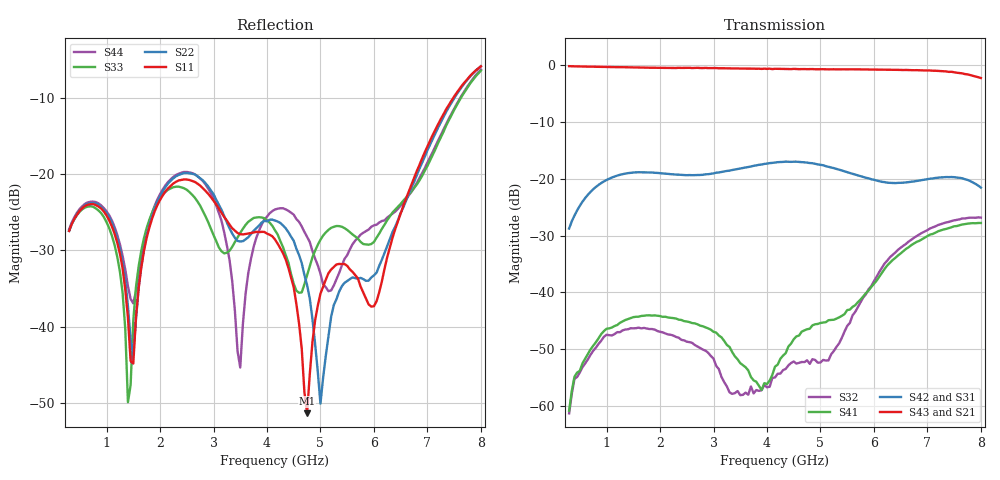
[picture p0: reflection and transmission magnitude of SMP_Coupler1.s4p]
! Created Sat Oct 21 10:14:57 2017
# hz S ma R 50
! 4 Port Network Data from SP1.SP block
! freq  magS11  angS11  magS12  angS12  magS13  angS13  magS14  angS14
!  magS21  angS21  magS22  angS22  magS23  angS23  magS24  angS24
!  magS31  angS31  magS32  angS32  magS33  angS33  magS34  angS34
!  magS41  angS41  magS42  angS42  magS43  angS43  magS44  angS44
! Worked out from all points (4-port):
!   155 points, 300 MHz to 8 GHz, reference 50 ohm
!   strongest paths, dB at 300 MHz, 2.2 GHz, 4.15 GHz, 6.1 GHz, 8 GHz:
!     S43: -0.1, -0.5, -0.6, -0.7, -2.2
!     S21: -0.1, -0.5, -0.6, -0.7, -2.4
!     S42: -28.8, -19.2, -17.1, -20.4, -21.6
!     S31: -28.8, -19.2, -17.1, -20.3, -21.0
!     S41: -60.9, -44.5, -53.1, -37.3, -27.8
!     S32: -61.4, -47.5, -55.0, -36.4, -26.8
!   lowest |S11| = -51.4 dB at 4.75 GHz (marker M1), VSWR 1.01, Z = 49.7 - j0.0107 ohm
!   |S11| at or under -10 dB: start of sweep to 7.481 GHz
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3e8  0.04244 27.7  0.9831 -40.6  0.03636 48.3  0.0009341 115.9
     0.9838 -40.4  0.04276 28.2  0.0008734 116.6  0.03641 48.6
     0.0363 48.6  0.0008558 114.7  0.0424 29.4  0.9844 -40.4
     0.0009028 116.1  0.03646 48.7  0.9841 -40.4  0.04352 27.7
1.3e9  0.02411 -120.5  0.9631 -173.1  0.11 -82.8  0.005552 -120.0
       0.9638 -173.1  0.02633 -125.2  0.004587 -121.2  0.1099 -83.3
       0.11 -82.8  0.004608 -121.1  0.01668 -111.2  0.9629 -172.7
       0.005533 -120.5  0.1099 -83.2  0.9637 -172.7  0.02914 -139.8
2.65e9  0.08906 -110.6  0.948 8.3  0.1076 99.9  0.005273 -23.3
        0.9498 8.4  0.09961 -116.2  0.003448 -7.6  0.1076 98.5
        0.1075 99.7  0.003423 -7.8  0.07016 -101.8  0.9478 9.2
        0.005314 -23.2  0.1077 98.7  0.9495 9.4  0.1001 -127.6
3.45e9  0.04116 -161.4  0.9392 -98.4  0.121 -6.7  0.002487 171.6
        0.9396 -98.3  0.03649 -164.6  0.001295 -108.4  0.1216 -9.2
        0.1208 -6.9  0.001345 -108.3  0.03842 -98.4  0.9367 -97.2
        0.002563 169.4  0.1219 -9.3  0.9399 -97.2  0.006884 69.4
4.75e9  0.002694 -177.7  0.9246 87.9  0.1384 -179.9  0.004856 165.2
        0.925 87.9  0.01875 106.9  0.002403 130.0  0.1385 177.6
        0.1382 -179.9  0.002511 127.8  0.02168 -114.7  0.9243 89.6
        0.004717 162.9  0.1388 177.7  0.9259 89.5  0.03883 104.9
6e9  0.0136 145.7  0.9199 -81.7  0.1005 12.0  0.01167 -1.8
     0.9215 -81.7  0.02167 161.0  0.01263 16.2  0.09824 6.6
     0.1001 11.9  0.01251 15.9  0.03591 -162.8  0.9203 -79.5
     0.01186 -1.9  0.09803 6.7  0.9206 -79.6  0.04619 160.2
8e9  0.5111 -95.7  0.7586 -3.7  0.08856 85.9  0.0411 11.4
     0.7583 -3.4  0.512 -97.6  0.04568 11.2  0.0839 82.3
     0.08873 85.5  0.04547 10.9  0.4784 -93.3  0.7732 -2.1
     0.04079 11.6  0.08366 82.7  0.7738 -1.9  0.4861 -98.0
